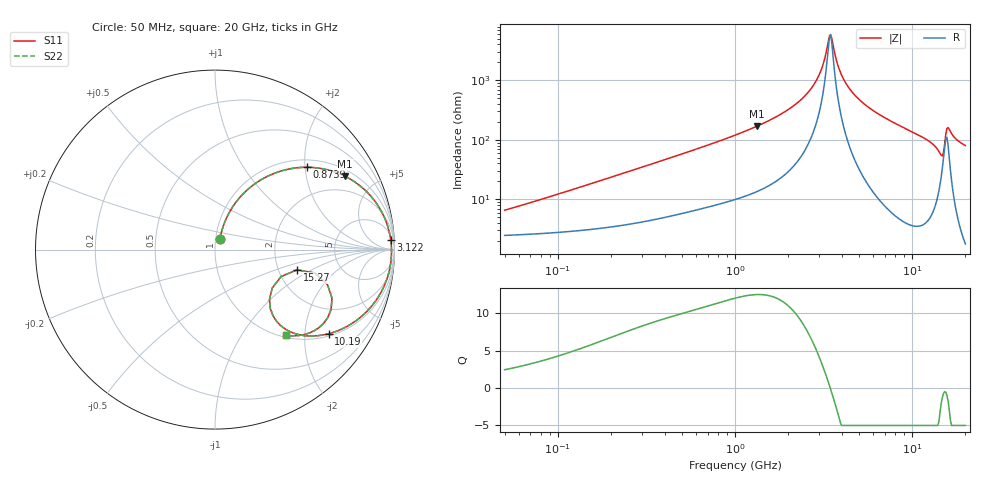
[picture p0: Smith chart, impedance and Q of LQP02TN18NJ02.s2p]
!Murata Part Number: LQP02TN18NJ02
!These Parameters are Measured in Series Mode Connection
!  o--[Z]--o
!Port1  Port2
!  o-------o
!Freq. Start=50[MHz] Stop=20[GHz], 401[Steps]
# Hz S RI R 50
!Freq.(Hz) S11(Real) S11(Imag) S21(Real) S21(Imag) S12(Real) S12(Imag) S22(Real) S22(Imag)
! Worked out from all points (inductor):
!   401 points, 50 MHz to 20 GHz, reference 50 ohm
!   read as one part in series: L = 19 nH near 64.5 MHz
!   highest Q = 12.5 at 1.329 GHz (marker M1), where L = 20.2 nH
!   self-resonance near 3.415 GHz
!   S11 on the Smith chart (normalised r, x): 50 MHz: 1.05, +0.12; 873.9 MHz: 1.18, +2.05; 3.122 GHz: 12, +33; 10.19 GHz: 1.07, -2.65; 15.27 GHz: 2.53, -0.73; 20 GHz: 1.04, -1.60
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5e7  0.0275 0.0576  0.9725 -0.0576  0.9725 -0.0576  0.0275 0.0576
1.364002e8  0.0523 0.1479  0.9477 -0.1479  0.9477 -0.1479  0.0523 0.1479
3.721004e8  0.182 0.3345  0.818 -0.3345  0.818 -0.3345  0.182 0.3345
8.738837e8  0.5126 0.4588  0.4874 -0.4588  0.4874 -0.4588  0.5126 0.4588
1e9  0.5815 0.4535  0.4185 -0.4535  0.4185 -0.4535  0.5815 0.4535
1.329223e9  0.7254 0.4081  0.2746 -0.4081  0.2746 -0.4081  0.7254 0.4081
2.05233e9  0.9004 0.2565  0.0996 -0.2565  0.0996 -0.2565  0.9004 0.2565
2.728004e9  0.9648 0.1215  0.0352 -0.1215  0.0352 -0.1215  0.9648 0.1215
3.121702e9  0.9794 0.0525  0.0206 -0.0525  0.0206 -0.0525  0.9794 0.0525
3.364474e9  0.9829 0.0135  0.0171 -0.0135  0.0171 -0.0135  0.9829 0.0135
3.466789e9  0.9835 -0.0022  0.0165 0.0022  0.0165 0.0022  0.9835 -0.0022
3.908127e9  0.9803 -0.0652  0.0197 0.0652  0.0197 0.0652  0.9803 -0.0652
4.405649e9  0.9685 -0.128  0.0315 0.128  0.0315 0.128  0.9685 -0.128
5.433528e9  0.9268 -0.2348  0.0732 0.2348  0.0732 0.2348  0.9268 -0.2348
7.442007e9  0.8119 -0.376  0.1881 0.376  0.1881 0.376  0.8119 -0.376
1.019291e10  0.6334 -0.4686  0.3666 0.4686  0.3666 0.4686  0.6334 -0.4686
1.334722e10  0.4006 -0.4482  0.5994 0.4482  0.5994 0.4482  0.4006 -0.4482
1.460232e10  0.3034 -0.2789  0.6966 0.2789  0.6966 0.2789  0.3034 -0.2789
1.527346e10  0.4569 -0.1127  0.5431 0.1127  0.5431 0.1127  0.4569 -0.1127
1.621653e10  0.6467 -0.3342  0.3533 0.3342  0.3533 0.3342  0.6467 -0.3342
1.747767e10  0.5311 -0.4623  0.4689 0.4623  0.4689 0.4623  0.5311 -0.4623
2e10  0.3931 -0.4775  0.6069 0.4775  0.6069 0.4775  0.3931 -0.4775
